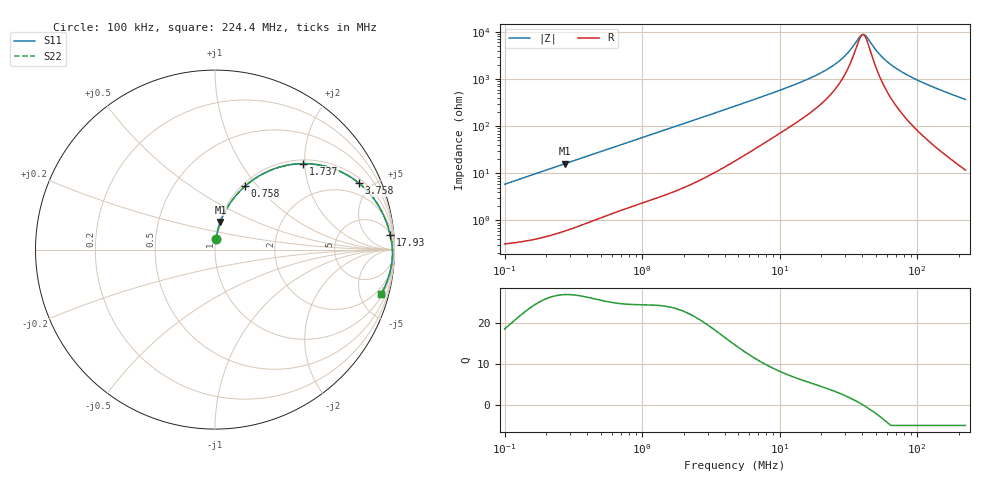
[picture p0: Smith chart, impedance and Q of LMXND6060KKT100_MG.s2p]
! LMXND6060KKT100_MG  S-PARAMETER MODEL  ( General Type )
! Model Generated by TAIYO YUDEN Corporation (https://www.yuden.co.jp/en/)
! Version 1.0
! TAIYO YUDEN Control No. 191023NI43SB-FBB
! Copyright(c) 2019 TAIYO YUDEN CO.,LTD. All Rights Reserved.
! Product Description (link to TY-COMPAS)
! https://ds.yuden.co.jp/TYCOMPAS/or/detail?pn=LMXND6060KKT100MMG&u=M
! Products Name : Inductors
! Characteristics :
!  Inductance : 10 uH , SRF(min) : 25 MHz , DC Resistance(max) : 0.324 Ohm
!  Rated Current : Saturation :1000 mA , Temp Rise : 1100 mA (40 degC)
!  Case Size : 6.0 x 6.0 / 0.236 x 0.236 [mm/inch] , Thickness : 1 / 0.039 [mm/inch]
!  (Conditions: Temperature = 25 degC , DC Bias Current/Voltage = 0A / 0V)
! External Node Assignments :
!  1  o---GGG---o  2
! GND o---------o GND
! Frequency Range : 0.1MHz  -  224.402193MHz  [ 402 STEP ]
# MHz S RI R 50
! Freq[MHz].  S11 Real  S11 Imag  S21 Real  S21 Imag  S12 Real  S12 Imag  S22 Real  S22 Imag
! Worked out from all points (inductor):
!   401 points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, 100 kHz to 224.4 MHz, reference 50 ohm
!   read as one part in series: L = 9.33 uH near 103.9 kHz
!   highest Q = 26.8 at 272.7 kHz (marker M1), where L = 9.29 uH
!   self-resonance near 39.54 MHz
!   S11 on the Smith chart (normalised r, x): 100 kHz: 1.01, +0.12; 758 kHz: 1.04, +0.87; 1.737 MHz: 1.08, +1.96; 3.758 MHz: 1.25, +4.21; 17.93 MHz: 6, +23; 224.4 MHz: 1.23, -7.37
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0.1  0.00657 0.0581  0.9934 -0.0581  0.9934 -0.0581  0.00657 0.0581
0.272668  0.0302 0.1534  0.9698 -0.1534  0.9698 -0.1534  0.0302 0.1534
0.364164  0.0498 0.1995  0.9502 -0.1995  0.9502 -0.1995  0.0498 0.1995
0.757957  0.1682 0.3542  0.8318 -0.3542  0.8318 -0.3542  0.1682 0.3542
1.326154  0.3653 0.4612  0.6347 -0.4612  0.6347 -0.4612  0.3653 0.4612
1.737321  0.4897 0.479  0.5103 -0.479  0.5103 -0.479  0.4897 0.479
2.458534  0.6495 0.4542  0.3505 -0.4542  0.3505 -0.4542  0.6495 0.4542
3.758225  0.803 0.3695  0.197 -0.3695  0.197 -0.3695  0.803 0.3695
4.737111  0.8603 0.314  0.1397 -0.314  0.1397 -0.314  0.8603 0.314
8.129905  0.9367 0.1969  0.0633 -0.1969  0.0633 -0.1969  0.9367 0.1969
17.25085  0.9755 0.0859  0.0245 -0.0859  0.0245 -0.0859  0.9755 0.0859
17.9294  0.9766 0.0815  0.0234 -0.0815  0.0234 -0.0815  0.9766 0.0815
27.40768  0.9851 0.0371  0.0149 -0.0371  0.0149 -0.0371  0.9851 0.0371
31.98105  0.987 0.0221  0.013 -0.0221  0.013 -0.0221  0.987 0.0221
38.04441  0.9885 0.00552  0.0115 -0.00552  0.0115 -0.00552  0.9885 0.00552
40.311  0.9888 -3.68e-05  0.0112 3.68e-05  0.0112 3.68e-05  0.9888 -3.68e-05
42.71263  0.989 -0.00562  0.011 0.00562  0.011 0.00562  0.989 -0.00562
52.80919  0.9891 -0.0266  0.0109 0.0266  0.0109 0.0266  0.9891 -0.0266
62.8214  0.9883 -0.0448  0.0117 0.0448  0.0117 0.0448  0.9883 -0.0448
77.67135  0.986 -0.0688  0.014 0.0688  0.014 0.0688  0.986 -0.0688
103.7348  0.9796 -0.1065  0.0204 0.1065  0.0204 0.1065  0.9796 -0.1065
224.4022  0.9246 -0.2487  0.0754 0.2487  0.0754 0.2487  0.9246 -0.2487
